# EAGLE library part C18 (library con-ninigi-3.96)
NINIGI
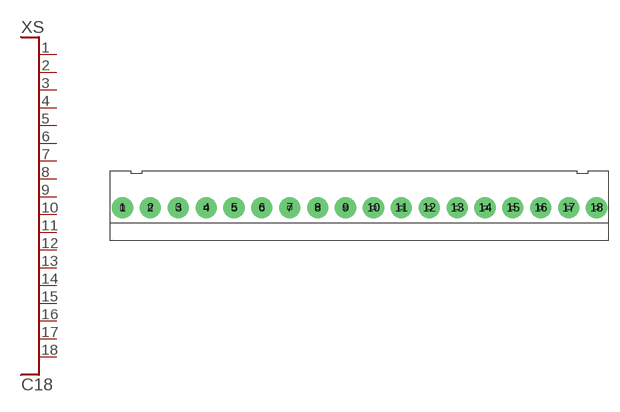
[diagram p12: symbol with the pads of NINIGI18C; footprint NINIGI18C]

Designator prefix XS

## C18  [NINIGI18C]
1  P$1
2  P$2
3  P$3
4  P$4
5  P$5
6  P$6
7  P$7
8  P$8
9  P$9
10  P$10
11  P$11
12  P$12
13  P$13
14  P$14
15  P$15
16  P$16
17  P$17
18  P$18

## Footprint NINIGI18C (pad centres in mm)
drill 1.6 pad 3: 1 -33.66,0; 2 -29.7,0; 3 -25.74,0; 4 -21.78,0; 5 -17.82,0; 6 -13.86,0; 7 -9.9,0; 8 -5.94,0; 9 -1.98,0; 10 1.98,0; 11 5.94,0; 12 9.9,0; 13 13.86,0; 14 17.82,0; 15 21.78,0; 16 25.74,0; 17 29.7,0; 18 33.66,0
